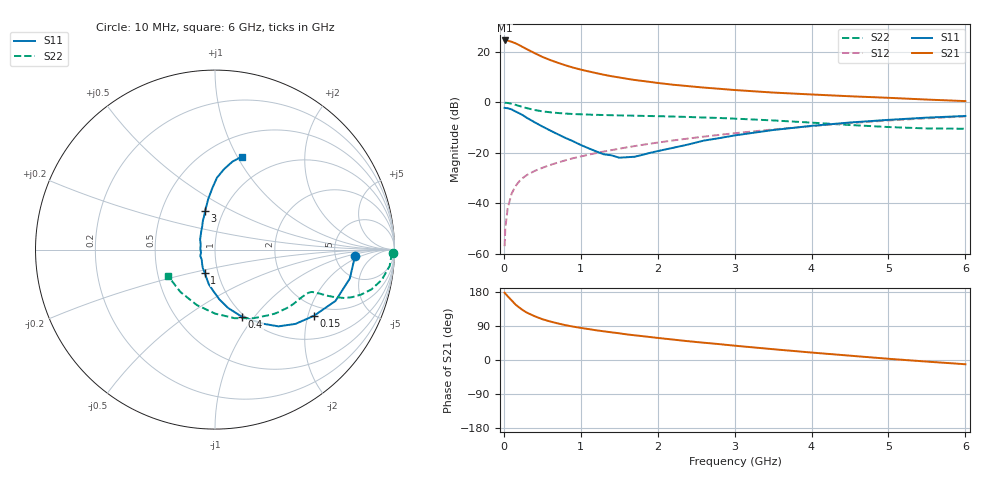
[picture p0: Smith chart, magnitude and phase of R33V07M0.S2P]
! SIEMENS Small Signal Semiconductors
! BFR181
! Si NPN RF Bipolar Junction Transistor in SOT23
! VCE = 3 V  IC = 7 mA
! Common Emitter S-Parameters:  May  1996
# GHz  S  MA  R  50
!  f  S11  S21  S12  S22
! GHz  MAG  ANG  MAG  ANG  MAG  ANG  MAG  ANG
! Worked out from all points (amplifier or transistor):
!   36 points, 10 MHz to 6 GHz, reference 50 ohm
!   highest |S21| = 24.6 dB at 10 MHz (marker M1)
!   |S21| within 3 dB of that: start of sweep to 269.9 MHz
!   unconditionally stable (mu >= 1): 934.1 MHz to 2.773 GHz
!   at 250 MHz: K = 0.51, MSG = 25.9 dB, |S12| = -29.9 dB
!   at 1.4 GHz: K = 1.06, MAG = 13.2 dB, |S12| = -18.9 dB
!   at 6 GHz: K = 0.86, MSG = 3.0 dB, |S12| = -5.6 dB
!   S11 on the Smith chart (normalised r, x): 10 MHz: 7.90, -1.38; 150 MHz: 1.66, -2.19; 400 MHz: 0.97, -0.87; 1 GHz: 0.86, -0.23; 3 GHz: 0.82, +0.37; 6 GHz: 0.71, +1.04
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0.01  0.7813 -2.5  17.03 177.5  0.0014 98.9  0.9893 -1.1
0.02  0.7759 -4.9  16.95 175.0  0.0033 86.2  0.9832 -2.2
0.05  0.7683 -12.1  16.92 168.2  0.0079 84.7  0.9772 -5.4
0.1  0.7295 -23.1  16.04 157.6  0.0153 77.7  0.9443 -10.3
0.15  0.6637 -33.7  14.99 146.7  0.0216 73.6  0.8991 -14.3
0.2  0.6103 -42.7  13.78 138.5  0.0271 70.3  0.8519 -17.1
0.25  0.5551 -50.4  12.51 131.1  0.0319 68.3  0.8093 -19.1
0.3  0.4941 -56.8  11.4 124.9  0.0363 67.3  0.7707 -20.5
0.4  0.4045 -68.0  9.549 115.6  0.0436 65.8  0.7088 -21.8
0.5  0.3337 -77.3  8.044 107.7  0.0503 65.7  0.6663 -22.5
0.6  0.2788 -84.9  6.981 101.7  0.0572 66.1  0.6386 -22.7
0.8  0.1978 -99.8  5.471 92.0  0.071 66.3  0.6016 -23.3
1  0.1431 -113.3  4.492 84.8  0.0844 67.3  0.5811 -24.1
1.1  0.1232 -123.5  4.142 81.6  0.0918 67.3  0.5739 -24.8
1.3  0.0933 -142.1  3.552 75.7  0.1062 67.2  0.5627 -26.3
1.6  0.0817 177.5  2.952 67.5  0.1285 66.7  0.5499 -29.2
2.2  0.1257 127.8  2.249 53.9  0.1761 64.4  0.5248 -36.7
3  0.2215 104.4  1.766 37.8  0.245 58.8  0.4772 -49.6
3.5  0.2835 97.7  1.573 28.5  0.2909 54.5  0.4396 -60.3
4.5  0.4 88.5  1.327 11.4  0.3891 43.8  0.3567 -89.9
5.5  0.4996 78.8  1.141 -4.2  0.4842 31.0  0.3047 -129.3
6  0.539 74.0  1.064 -11.2  0.5278 24.0  0.3006 -151.1
